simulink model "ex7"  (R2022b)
settings: Solver=ode45  StartTime=0.0  StopTime=10.0  RelTol=1e-3  EnableMultiTasking=on

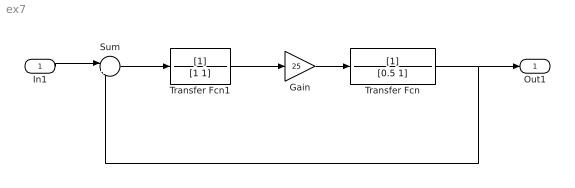
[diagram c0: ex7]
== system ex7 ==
  In1 : Inport
  Gain : Gain  Gain=25
  Sum : Sum  Inputs=|+-
  Transfer Fcn : TransferFcn  Denominator=[0.5 1]
  Transfer Fcn1 : TransferFcn  Denominator=[1 1]
  Out1 : Outport
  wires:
  Transfer Fcn1/1 -> Gain/1
  Gain/1 -> Transfer Fcn/1
  Sum/1 -> Transfer Fcn1/1
  In1/1 -> Sum/1
  Transfer Fcn/1 -> Sum/2, Out1/1
